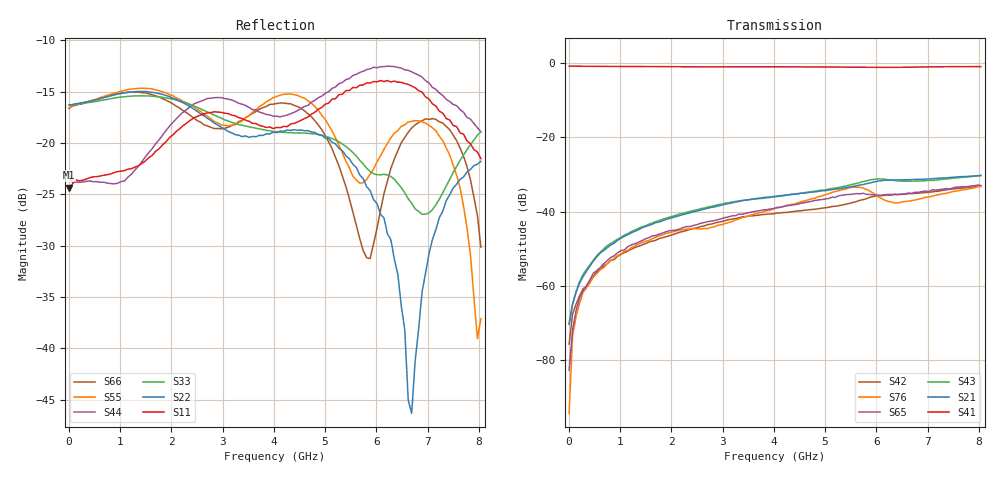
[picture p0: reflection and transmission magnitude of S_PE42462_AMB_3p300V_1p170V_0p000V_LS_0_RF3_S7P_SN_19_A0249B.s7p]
! Device ID: PE42462
! File Path: z:\PE42462\DataSheet S-parameter-6T\AMB\3p300\LS_0_RF3\PE42462_AMB_3p300V_1p170V_0p000V_LS_0_RF3_S7P_SN_19_A0249B.s7p
! Serial: 19
! Lot: A0249B
! Temp: AMB
! VDD: 3.300
! VSS: 0.000
! Control_Hi: 1.170
! Control_Lo: 0.000
! Logic State: LS_0_RF3
! Port 1:
! Port 2:
! Port 3:
! Port 4:
! Port 5:
! Port 6:
! Port 7:
! ThroughPath:1-4
! IDD: 0.0001058258
! ISS/IDD2: -1.67e-008
! IDMM3/IDD3: -2.028e-007
! Comment:
#  Hz  S  RI  R  50
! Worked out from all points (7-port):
!   120 points, 10 MHz to 8.037 GHz, reference 50 ohm
!   strongest paths, dB at 10 MHz, 2.034 GHz, 4.057 GHz, 6.08 GHz, 8.037 GHz:
!     S41: -0.8, -0.9, -0.9, -1.1, -0.9
!     S21: -70.5, -41.6, -35.9, -31.7, -30.3
!     S43: -70.2, -41.3, -36.0, -31.2, -30.3
!     S65: -82.9, -45.1, -38.9, -35.8, -33.0
!     S76: -94.5, -45.5, -39.0, -36.4, -33.2
!     S42: -75.8, -46.2, -40.4, -35.6, -33.1
!   lowest |S11| = -24.3 dB at 10 MHz (marker M1), VSWR 1.13, Z = 56.5 - j0.215 ohm
!   |S11| at or under -10 dB: start of sweep to end of sweep
